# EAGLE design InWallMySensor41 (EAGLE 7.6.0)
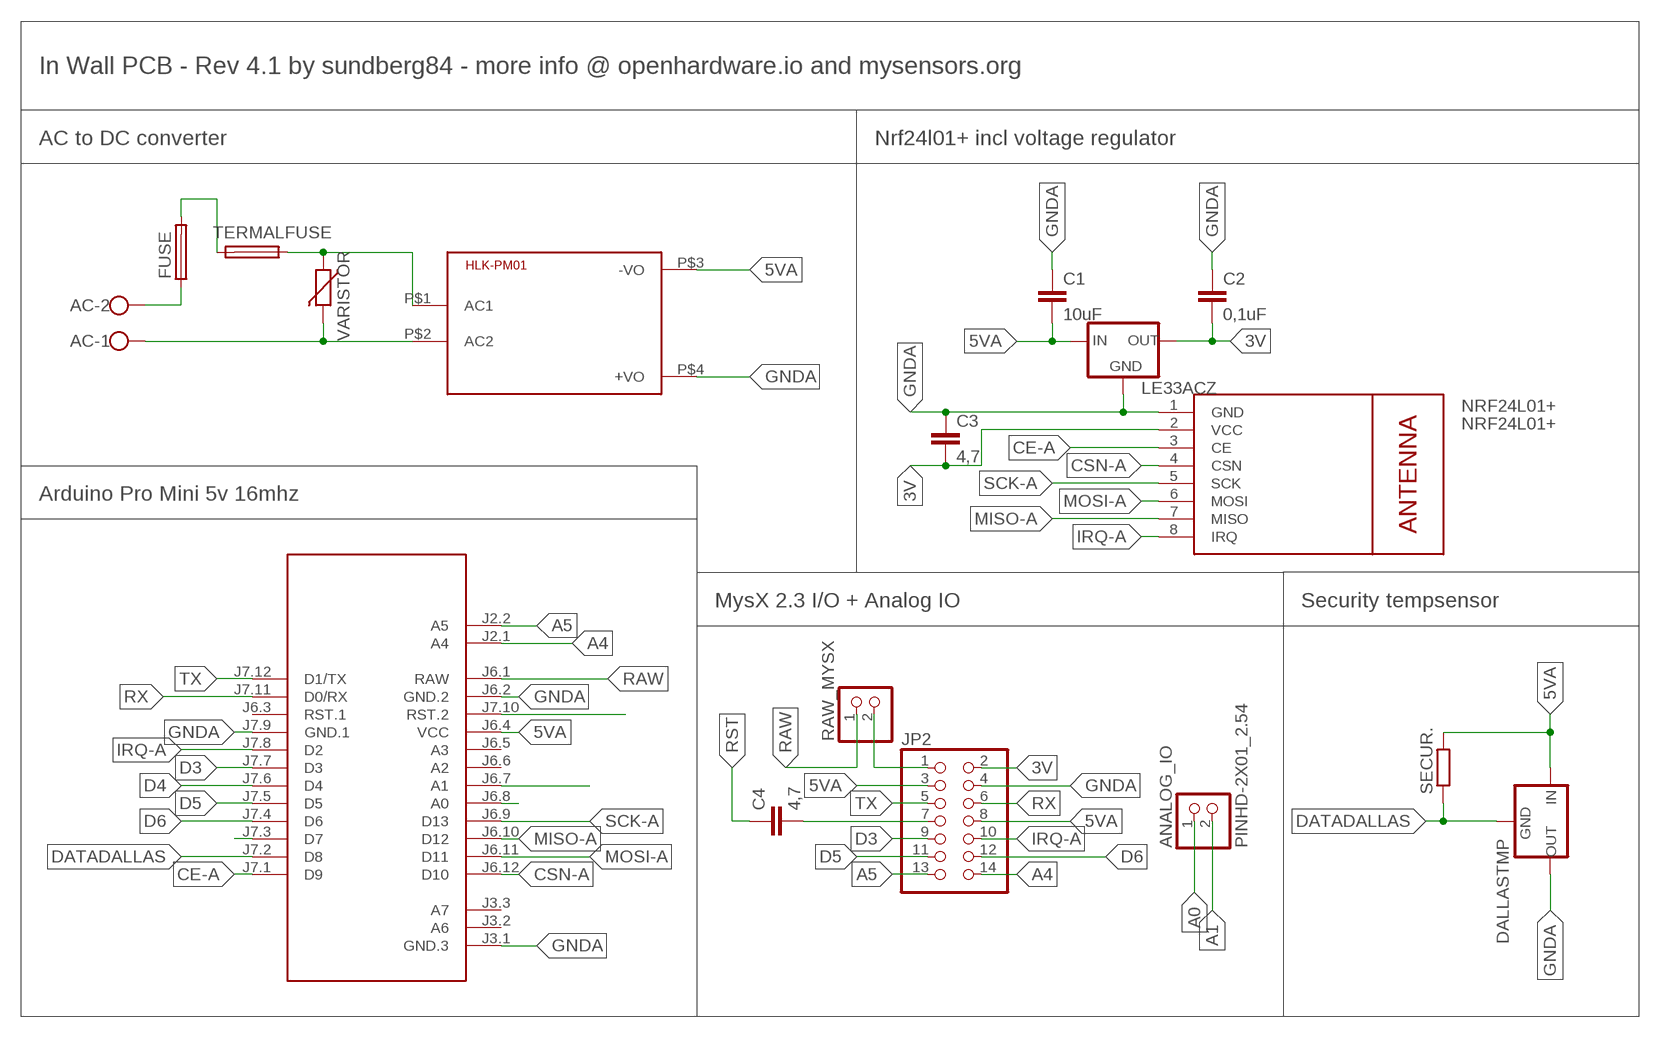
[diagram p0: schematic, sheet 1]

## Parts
AC  W237-102  [W237-102]
ANALOG_IO  PINHD-2X01_2.54  [2X01]
C1  10uF  C5/2.5  [C5B2.5]
C2  0,1uF  C5/2.5  [C5B2.5]
C3  4,7  C5/2.5  [C5B2.5]
C4  4,7  C5/2.5  [C5B2.5]
DALLASTMP  78LXX  [78LXX]
FUSE  FUSETE5  [TE5]
HLK-PM01  HKLPM01  [HKLPM01]
JP2  PINHD-2X07_2.54  [2X07]
LE33ACZ  78LXX  [78LXX]
M1  ARDUINO-PRO-MINI-3.3V#NP  [ARDUINO-PRO-MINI#NP]
NRF24L01+  NRF24L01+  WIRELESS-NRF24L01  [WIRELESS-NRF24L01]
RAW_MYSX  PINHD-1X02_2.54-S  [1X02-S]
SECUR.  R-EU_0204/5  [0204/5]
TERMALFUSE  FUSETE5  [TE5]
VARISTOR  VARISTOR-7,5  [R-7,5]

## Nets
3V: C2.2 C3.2 JP2.2 LE33ACZ.OUT NRF24L01+.2(VCC)
5VA: C1.2 DALLASTMP.IN HLK-PM01.P$3(-VO) JP2.3 JP2.8 LE33ACZ.IN M1.J6.4(VCC) SECUR..2
A0: ANALOG_IO.1 M1.J6.8(A0)
A1: ANALOG_IO.2 M1.J6.7(A1)
A4: JP2.14 M1.J2.1(A4)
A5: JP2.13 M1.J2.2(A5)
ACGND: AC.1 HLK-PM01.P$2(AC2) VARISTOR.2
CE-A: M1.J7.1(D9) NRF24L01+.3(CE)
CSN-A: M1.J6.12(D10) NRF24L01+.4(CSN)
D3: JP2.9 M1.J7.7(D3)
D4: M1.J7.6(D4)
D5: JP2.11 M1.J7.5(D5)
D6: JP2.12 M1.J7.4(D6)
D7: M1.J7.3(D7)
DATADALLAS: DALLASTMP.GND M1.J7.2(D8) SECUR..1
GNDA: C1.1 C2.1 C3.1 DALLASTMP.OUT HLK-PM01.P$4(+VO) JP2.4 LE33ACZ.GND M1.J3.1(GND.3) M1.J6.2(GND.2) M1.J7.9(GND.1) NRF24L01+.1(GND)
IRQ-A: JP2.10 M1.J7.8(D2) NRF24L01+.8(IRQ)
MISO-A: M1.J6.10(D12) NRF24L01+.7(MISO)
MOSI-A: M1.J6.11(D11) NRF24L01+.6(MOSI)
N$1: FUSE.2 TERMALFUSE.2
N$4: AC.2 FUSE.1
N$6: JP2.1 RAW_MYSX.2
N$7: HLK-PM01.P$1(AC1) TERMALFUSE.1 VARISTOR.1
N$8: C4.2 JP2.7
RAW: M1.J6.1(RAW) RAW_MYSX.1
RST: C4.1 M1.J7.10(RST.2)
RX: JP2.6 M1.J7.11(D0/RX)
SCK-A: M1.J6.9(D13) NRF24L01+.5(SCK)
TX: JP2.5 M1.J7.12(D1/TX)
Unconnected: M1.J3.2(A6) M1.J3.3(A7) M1.J6.3(RST.1) M1.J6.5(A3) M1.J6.6(A2)

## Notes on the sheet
- In Wall PCB - Rev 4.1 by sundberg84 - more info @ openhardware.io and mysensors.org
- AC to DC converter | Nrf24l01+ incl voltage regulator
- Arduino Pro Mini 5v 16mhz
- MysX 2.3 I/O + Analog IO | Security tempsensor

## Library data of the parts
AC = con-wago-500:W237-102: WAGO SCREW CLAMP; MPN: 237-102; OC_FARNELL: unknown; OC_NEWARK: 70K9898
ANALOG_IO = pinhead-2:PINHD-2X01
C1-C4 = capacitor-wima:C: CAPACITOR
DALLASTMP LE33ACZ = v-reg:78LXX: VOLTAGE REGULATOR
FUSE TERMALFUSE = fuse:FUSE: Fuse; OC_FARNELL: unknown; OC_NEWARK: unknown
HLK-PM01 = HKLPM01:HKLPM01
JP2 = pinhead-2:PINHD-2X07: PIN HEADER
M1 = diy-modules:ARDUINO-PRO-MINI-*#NP: Arduino Pro Mini without programming pads
NRF24L01+ = diy-modules:WIRELESS-NRF24L01: 2.4 GHz Wireless Module based on NRF24L01 chip
RAW_MYSX = pinhead-2:PINHD-1X02: PIN HEADER
SECUR. = resistor:R-EU_: RESISTOR, European symbol
VARISTOR = varistor:VARISTOR: VARISTOR

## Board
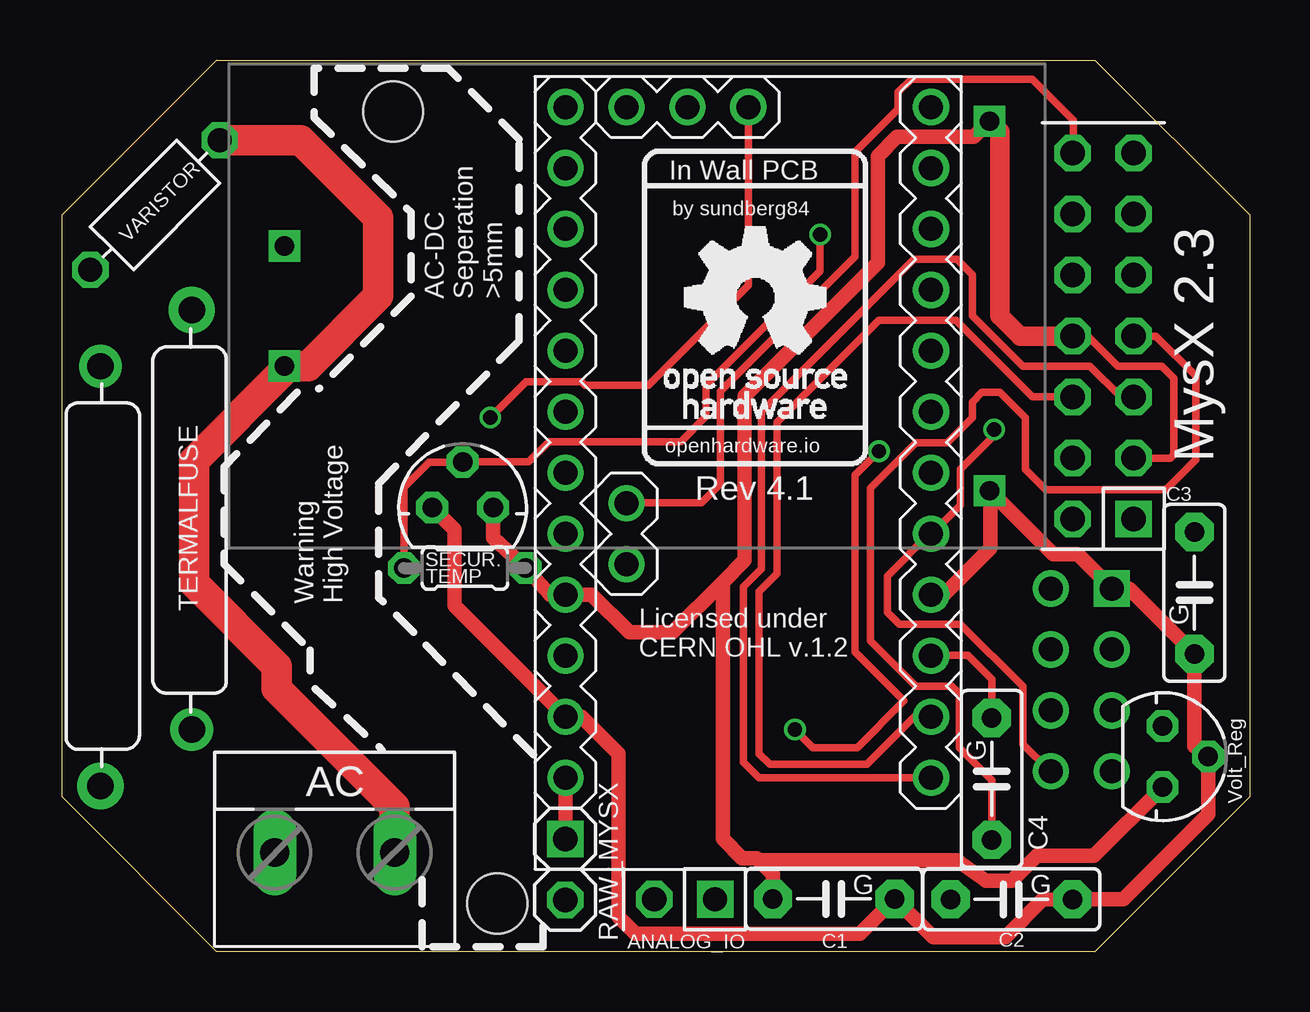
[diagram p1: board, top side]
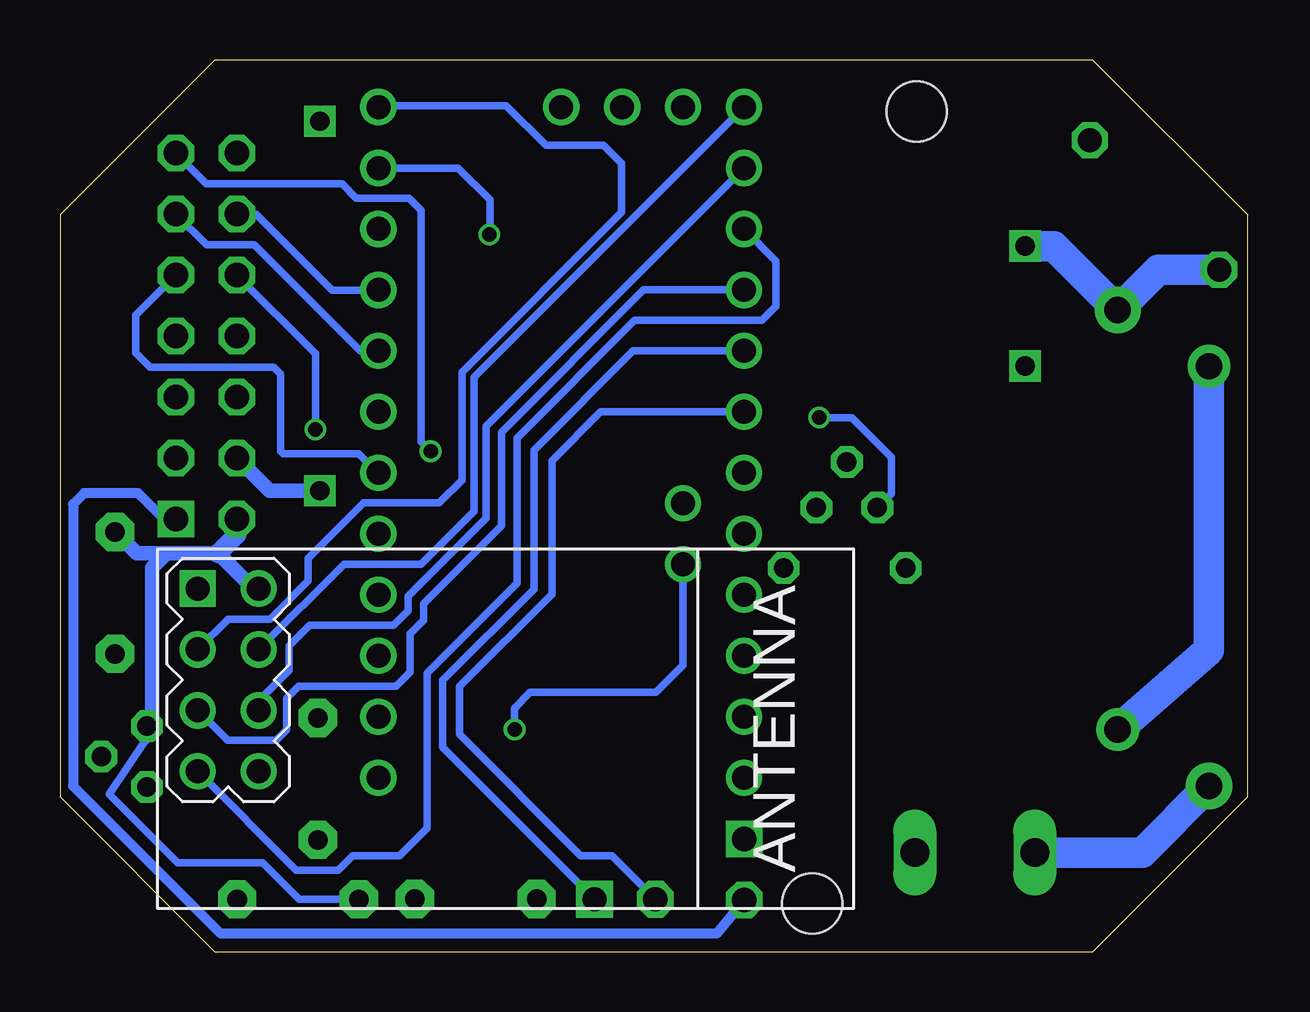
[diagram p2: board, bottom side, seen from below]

Size 49.5 x 37.15 mm. Coordinates in mm from the lower left corner, seen from the top.
Outline: 6.45,37.15 43.05,37.15 49.5,30.7 49.5,6.45 43.05,0 6.45,0 0,6.45 0,30.7 6.45,37.15
Copper layers (1*16): Top 0.035mm / dielectric 1.5mm / Bottom 0.035mm
Design rules "ITead_rule": minimum track width 6mil, minimum drill 12mil, track to track 6mil, track to pad 6mil, pad to pad 6mil, via to via 6mil, smd to smd 0mil, copper to edge 10mil, drill to drill 10mil, minimum pad ring 10mil, minimum via ring 6mil, stop-mask expansion 2mil, vias tented up to drill 100mil, thermal gap 10mil
Holes 2.5 mm at 18.15,2 13.8,35

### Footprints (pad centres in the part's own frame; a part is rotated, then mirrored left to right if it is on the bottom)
W237-102 = drill 1.194 long: 1 -2.5,-1.27; 2 2.5,-1.27
2X01 = drill 1.016 square: 1 -1.27,-1.27 | drill 1.016 octagon: 2 -1.27,1.27
C5B2.5 = drill 0.813 pad 1.6 octagon: 1 -2.54,0; 2 2.54,0
78LXX = drill 0.813 octagon: GND 0,1.905; IN 1.27,0; OUT -1.27,0
TE5 = drill 1.1 pad 1.93: 1 -5.632,0 | drill 1.1 pad 1.778: 2 11.852,0
HKLPM01 = drill 0.8 square: P$1 -14.7,2.5; P$2 -14.7,-2.5; P$3 14.7,7.7; P$4 14.7,-7.7
2X07 = drill 1.016 square: 1 -7.62,-1.27 | drill 1.016 octagon: 2 -7.62,1.27; 3 -5.08,-1.27; 4 -5.08,1.27; 5 -2.54,-1.27; 6 -2.54,1.27; 7 0,-1.27; 8 0,1.27; 9 2.54,-1.27; 10 2.54,1.27; 11 5.08,-1.27; 12 5.08,1.27; 13 7.62,-1.27; 14 7.62,1.27
ARDUINO-PRO-MINI#NP = drill 1: J2.1 -1.27,5.08; J2.2 -3.81,5.08; J3.1 15.24,0; J3.2 15.24,2.54; J3.3 15.24,5.08; J6.1 -12.7,7.62; J6.2 -10.16,7.62; J6.3 -7.62,7.62; J6.4 -5.08,7.62; J6.5 -2.54,7.62; J6.6 0,7.62; J6.7 2.54,7.62; J6.8 5.08,7.62; J6.9 7.62,7.62; J6.10 10.16,7.62; J6.11 12.7,7.62; J6.12 15.24,7.62; J7.1 15.24,-7.62; J7.2 12.7,-7.62; J7.3 10.16,-7.62; J7.4 7.62,-7.62; J7.5 5.08,-7.62; J7.6 2.54,-7.62; J7.7 0,-7.62; J7.8 -2.54,-7.62; J7.9 -5.08,-7.62; J7.10 -7.62,-7.62; J7.11 -10.16,-7.62; J7.12 -12.7,-7.62
WIRELESS-NRF24L01 = drill 1 square: 1 -12.7,6.35 | drill 1: 2 -10.16,6.35; 3 -12.7,3.81; 4 -10.16,3.81; 5 -12.7,1.27; 6 -10.16,1.27; 7 -12.7,-1.27; 8 -10.16,-1.27
1X02-S = drill 1.016 square: 1 -1.27,0 | drill 1.016 octagon: 2 1.27,0
0204/5 = drill 0.813 octagon: 1 -2.54,0; 2 2.54,0
R-7,5 = drill 1 octagon: 1 -3.81,0; 2 3.81,0

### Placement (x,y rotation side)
AC  11.37,2.85 180 top
ANALOG_IO  25.95,3.45 90 top
C1  32.17,2.2 180 top
C2  39.57,2.18 180 top
C3  47.2,14.95 90 top
C4  38.75,7.2 270 top
DALLASTMP  16.7,18.5 0 top
FUSE  1.61,12.54 90 top
HLK-PM01  23.97,26.9 0 top
JP2  43.4,25.65 90 top
LE33ACZ  45.87,8.12 270 top
M1  28.61,19.95 90 top
NRF24L01+  31.06,8.78 0 bottom
RAW_MYSX  20.98,3.43 270 top
SECUR.  16.79,15.98 0 top
TERMALFUSE  5.41,21.1 270 top
VARISTOR  3.88,31.11 45 top

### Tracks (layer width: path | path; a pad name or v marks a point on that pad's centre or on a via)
3V
  Bottom 0.305: 45.9,8.85 47.45,6.55 44.6,3.7 41.05,3.7 39.53,2.18 C2.2
  Bottom 0.406: 45.9,8.85 LE33ACZ.OUT
  Bottom 0.61: NRF24L01+.2 41.43,15.13 42.9,16.6 45.05,16.6 | 45.05,16.6 45.65,16 45.65,9.47 LE33ACZ.OUT | C3.2 46.31,16.6 45.05,16.6
  Bottom 0.813: JP2.2 42.13,17.37 42.9,16.6
5VA
  Top 0.305: 42.15,25.65 JP2.8 42.75,25.65 44,24.4 45.85,24.4 46.35,23.9 46.35,20.7 46.2,20.55 44.69,20.55 JP2.3
  Top 0.61: 27.55,15.4 28.45,16.3 28.45,23.15 34,28.7 34,33.15 34.8,33.95 38.02,33.95 HLK-PM01.P$3 | 27.55,15.4 27.55,4.7 28.35,3.9 28.95,3.9 29.07,3.78 | 27.55,15.4 25.45,13.3 23.65,13.3 22.08,14.87 M1.J6.4 20.34,14.87 SECUR..2 17.97,17.24 DALLASTMP.IN | C1.2 29.63,3.22 29.07,3.78 | 29.07,3.78 29.1,3.8 37.3,3.8 38.5,2.95 39.59,2.95 40.64,4 43.02,4 LE33ACZ.IN
  Top 0.813: JP2.8 39.95,25.65 39.1,26.5 39.1,34.17 HLK-PM01.P$3
A0
  Bottom 0.305: ANALOG_IO.1 33.55,8.51 33.55,11.3 29.75,15.1 29.75,20.9 25.62,25.03 M1.J6.8
A1
  Bottom 0.305: ANALOG_IO.2 26.5,4 27.8,4 32.85,9.05 32.85,11.05 29,14.9 29,20.45 26.96,22.49 M1.J6.7
A4
  Top 0.305: M1.J2.1 23.55,18.7 26.65,18.7 27.45,19.5 27.45,23.35 33.05,28.95 33.05,33.3 34.85,35.1 34.85,35.8 35.4,36.35 40.45,36.35 42.15,34.65 42.15,33.29 JP2.14
A5  (via drill 0.6)
  Top 0.305: v34.05,20.85 33.05,19.85 33.05,12.5 35.1,10.45 33.15,8.5 31.3,8.5 v30.55,9.25
  Bottom 0.305: v34.05,20.85 34.45,21.25 34.45,30.9 34.95,31.4 37.15,31.4 37.75,32 43.4,32 JP2.13 | M1.J2.2 23.53,11.92 24.65,10.8 29.9,10.8 30.55,10.15 v30.55,9.25
ACGND
  Top 1.27: VARISTOR.2 9.95,33.8 13.18,30.57 13.18,27.32 10.25,24.4 HLK-PM01.P$2 9.27,24.22 5.5,20.45 5.5,15.35 8.95,11.9 8.95,10.95 13.87,6.04 AC.1
CE-A
  Bottom 0.305: NRF24L01+.3 42.49,13.85 40.75,13.85 39.15,15.45 39.15,16.4 36.85,18.7 33.7,18.7 32.75,19.65 32.75,24.15 26.1,30.8 26.1,32.85 26.85,33.6 29.25,33.6 30.9,35.25 36.17,35.25 M1.J7.1
CSN-A
  Bottom 0.305: NRF24L01+.4 37.65,16.15 34.45,16.15 32.25,18.35 32.25,23.93 M1.J6.12
D3
  Bottom 0.305: JP2.9 46.35,26.51 46.35,24.95 45.75,24.35 40.6,24.35 40.3,24.05 40.3,20.85 40.2,20.75 37.05,20.75 36.25,19.95 M1.J7.7
D5
  Bottom 0.305: M1.J7.5 36.98,25.03 41.4,29.45 43.39,29.45 JP2.11
D6
  Bottom 0.305: M1.J7.4 36.25,27.55 38.15,27.55 41.33,30.73 JP2.12
DATADALLAS  (via drill 0.6)
  Top 0.305: v31.6,29.88 31.6,28.35 26.85,23.6 26.85,22.3 25.8,21.25 20.3,21.25 19.46,20.4 DALLASTMP.GND 15.3,20.4 14.25,19.35 SECUR..1
  Bottom 0.305: M1.J7.2 32.9,32.65 31.58,31.33 31.58,29.9 v31.6,29.88
GNDA  (via drill 0.6)
  Top 0.305: v17.85,22.25 19.35,23.75 21.65,23.75 21.8,23.6 24.45,23.6 28.61,27.76 M1.J3.1
  Top 0.61: DALLASTMP.OUT 16.36,17.57 16.36,14.41 M1.J6.2 21.66,9.79 23.2,8.25 23.2,1.45 23.9,0.75 33.27,0.75 C1.1 36.31,0.6 39.32,0.6 40.87,2.15 C2.1 44.23,2.18 47.78,5.73 LE33ACZ.GND 47.2,8.55 C3.1 44.48,15.13 NRF24L01+.1 43.76,15.14 42.35,16.55 41.32,16.55 HLK-PM01.P$4 38.7,19.17 38.7,16.8 36.77,14.87 M1.J7.9
  Bottom 0.305: v17.85,22.25 16.5,22.25 14.85,20.6 14.85,19.08 DALLASTMP.OUT
  Bottom 0.61: JP2.4 40.76,19.2 HLK-PM01.P$4
IRQ-A  (via drill 0.6)
  Top 0.305: v38.85,21.75 38.85,21.5 37.45,20.1 37.45,18.6 36.26,17.41 M1.J7.8 36.16,17.41 34.4,15.65 34.4,14.15 34.9,13.65 37.45,13.65 40.05,11.05 40.05,8.65 41.19,7.51 NRF24L01+.8
  Bottom 0.305: v38.85,21.75 38.85,24.91 JP2.10
MISO-A
  Bottom 0.305: M1.J6.10 19.65,28.77 19.65,26.9 20.25,26.3 25.55,26.3 30.45,21.4 30.45,15.35 34.2,11.6 34.2,5.15 35.35,4 37.3,4 37.9,3.4 39.65,3.4 NRF24L01+.7
MOSI-A
  Bottom 0.305: M1.J6.11 31.75,21.89 31.75,18.05 35,14.8 35,14.2 35.6,13.6 39.1,13.6 39.95,12.75 39.95,11.71 41.22,10.45 NRF24L01+.6
N$1
  Bottom 1.27: TERMALFUSE.2 1.61,12.55 FUSE.2
N$4
  Bottom 1.27: AC.2 4.39,4.12 FUSE.1
N$6
  Bottom 0.406: RAW_MYSX.2 22.13,0.75 42.8,0.75 48.95,6.9 48.95,18.65 48.5,19.1 46.25,19.1 45.18,18.03 JP2.1
N$7
  Bottom 1.27: VARISTOR.1 3.73,28.42 TERMALFUSE.1 8.08,29.4 HLK-PM01.P$1
N$8
  Top 0.305: JP2.7 45.6,25.65 47.25,24 47.25,20.5 46,19.25 41,19.25 40.15,20.1 40.15,22.25 39.1,23.3 38.35,23.3 37.95,22.9 37.95,22.25 36.9,21.2 35.6,21.2 33.7,19.3 33.7,12.95 35.6,11.05 37.1,11.05 37.4,10.75 37.4,8.5 38.75,7.15 C4.2
RAW
  Top 0.61: RAW_MYSX.1 20.99,5.83 M1.J6.1
RST
  Top 0.305: C4.1 38.75,11.35 37.75,12.35 36.25,12.35 M1.J7.10
RX
  Top 0.305: M1.J7.11 35.54,9.79 33.55,7.8 29.5,7.8 29.05,8.25 29.05,15 29.8,15.75 29.8,22.05 34.05,26.3 37.25,26.3 40.44,23.11 JP2.6
SCK-A
  Bottom 0.305: NRF24L01+.5 42.51,8.8 40.5,8.8 40.05,9.25 40.05,10.55 39.55,11.05 35.5,11.05 34.9,11.65 34.9,13.25 34.35,13.8 34.35,14.5 31.1,17.75 31.1,21.65 25.18,27.57 M1.J6.9
TX
  Top 0.305: M1.J7.12 29.05,7.25 28.4,7.9 28.4,15.2 29.15,15.95 29.15,22.5 35.5,28.85 37.3,28.85 37.95,28.2 37.95,26.5 40.05,24.4 42.85,24.4 44.14,23.11 JP2.5

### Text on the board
tPlace: In Wall PCB | by sundberg84 | AC-DC / Seperation / >5mm | openhardware.io | Rev 4.1 | Warning / High Voltage | Licensed under / CERN OHL v.1.2
tNames: MysX 2.3 | TEMP | G | G | Volt_Reg | G | G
